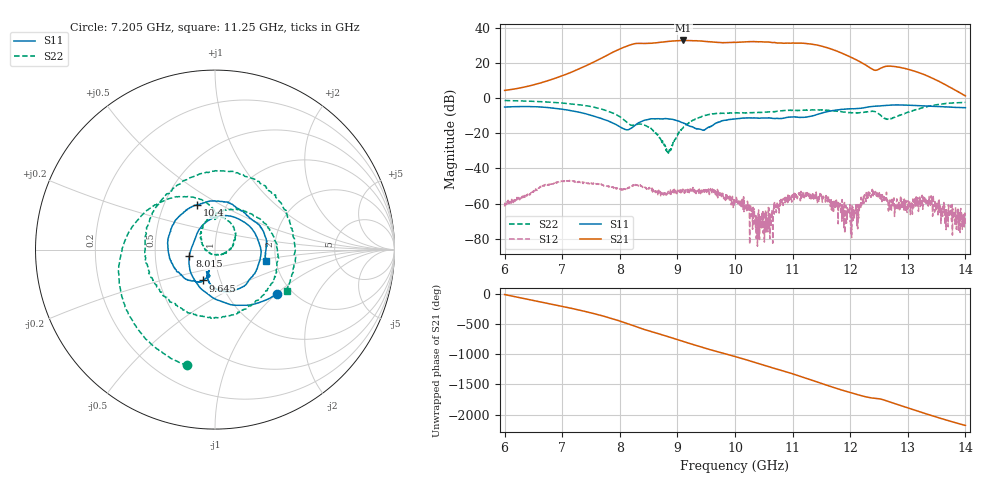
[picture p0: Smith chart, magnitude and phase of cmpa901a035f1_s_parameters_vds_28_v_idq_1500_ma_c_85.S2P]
!Keysight Technologies,E5071C,MY46110325,B.14.03
!Date: Wed Mar 10 14:13:47 2021
!Data & Calibration Information:
!Freq	S11:SOLT2(ON)	S21:SOLT2(ON)	S12:SOLT2(ON)	S22:SOLT2(ON)
!PortZ  Port1:50+j0  Port2:50+j0
!Above PortZ is port z conversion or system Z0 setting when saving the data.
!When reading, reference impedance value at option line is always used.
# Hz S dB R 50
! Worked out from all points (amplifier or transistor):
!   1601 points, 6 GHz to 14 GHz, reference 50 ohm
!   highest |S21| = 32.7 dB at 9.1 GHz (marker M1)
!   |S21| within 3 dB of that: 8.141 GHz to 11.47 GHz (3.334 GHz wide, 34 % of centre)
!   unconditionally stable (mu >= 1): start of sweep to end of sweep
!   at 7.33 GHz: K = 9.20, MAG = 19.9 dB, |S12| = -48.0 dB
!   at 10 GHz: K = 9.13, MAG = 32.6 dB, |S12| = -58.7 dB
!   at 14 GHz: K = 572.94, MAG = 6.3 dB, |S12| = -72.6 dB
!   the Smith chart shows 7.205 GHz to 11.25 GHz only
!   S11 on the Smith chart (normalised r, x): 7.205 GHz: 1.67, -1.00; 8.015 GHz: 0.75, -0.06; 9.645 GHz: 0.83, -0.29; 10.4 GHz: 0.73, +0.39; 11.25 GHz: 1.77, -0.25
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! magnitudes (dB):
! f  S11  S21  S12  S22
! 6 GHz  -5.1  4.3  -61.6  -1.4
! 6.67 GHz  -5.2  9.1  -49.7  -2.1
! 7.205 GHz  -7.5  15.3  -47.6  -3.6
! 7.335 GHz  -8.4  17.2  -48.3  -4.0
! 8.015 GHz  -16.6  28.1  -52.1  -10.9
! 8.67 GHz  -11.8  31.6  -53.6  -21.2
! 8.855 GHz  -11.9  32.2  -53.7  -30.2
! 9.1 GHz  -14.2  32.7  -52.8  -16.8
! 9.44 GHz  -18.2  32.3  -51.5  -10.3
! 9.645 GHz  -14.7  31.7  -53.1  -8.9
! 10 GHz  -11.9  31.7  -58.7  -8.4
! 10.19 GHz  -11.3  31.9  -61.3  -8.4
! 10.4 GHz  -11.4  32.0  -68.5  -8.1
! 10.62 GHz  -11.4  31.6  -72.8  -7.9
! 10.86 GHz  -11.3  31.1  -56.8  -7.1
! 11.25 GHz  -10.7  30.9  -53.7  -6.7
! 11.34 GHz  -10.3  30.6  -56.9  -6.7
! 12.04 GHz  -6.1  22.8  -63.7  -8.4
! 12.36 GHz  -4.9  17.0  -54.4  -7.6
! 12.67 GHz  -4.1  18.1  -59.8  -12.1
! 13.28 GHz  -4.5  13.4  -58.5  -5.4
! 14 GHz  -5.5  1.2  -72.6  -2.5
